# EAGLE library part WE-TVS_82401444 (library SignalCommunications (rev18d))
TVS Diode Super Speed Series Characteristics Operating temperature: –55 ºC to +85 °C for 824 014 x; –40 ºC to +85 °C for 824 016 46 Low clamping voltage Very low capacitance Rail to Rail protection Epoxy flame resistant UL94 V-0 RoHS, REACH and free of halogens Applications Super Speed data lines HDMI 1.3/1.4, DVI DisplayPort USB 3.0 SuperSpeed SATA GBit LAN ESD protection in accordance with EN 61000-4-2 – 8 kV contact discharge – 15 kV air discharge Updated by Dan Xu 2014-07-11 2014 (C) Wurth Elektronik
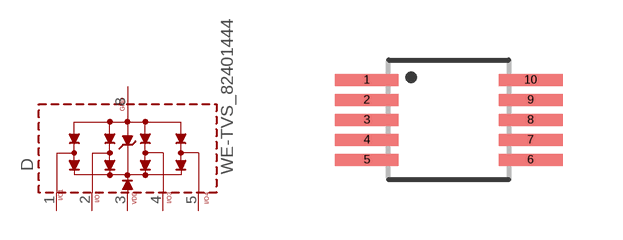
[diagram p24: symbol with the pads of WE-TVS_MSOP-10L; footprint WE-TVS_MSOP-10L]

Designator prefix D

## WE-TVS_82401444  [WE-TVS_MSOP-10L]
1  I/O1
2  I/O2
3  VDD  pwr
4  I/O3
5  I/O4
8  GND  pwr

## Footprint WE-TVS_MSOP-10L (pad centres in mm)
TVS Diode Array WE-TVS
smd 1.6 x 0.3: 1 -2.05,1; 2 -2.05,0.5; 3 -2.05,0; 4 -2.05,-0.5; 5 -2.05,-1; 6 2.05,-1; 7 2.05,-0.5; 8 2.05,0; 9 2.05,0.5; 10 2.05,1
